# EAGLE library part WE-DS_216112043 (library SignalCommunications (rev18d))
WE-DS D-SUB-Filter Connectors Bent 90° Characteristics Standard type filtered with 1000 pF High attenuation of more than 40 dB @ 180 MHz Choice of earthing metal sheet or high speed earthing clip Rated voltage: 100 VDC Rated current @ 20 ºC: 5 A Withstand voltage: 250 VRMS Insulation resistance: min. 1000 MΩ Operating temperature: –55 ºC to +125 ºC Applications Filtering of interfaces External connection to -printer -sensor -display Details see: http://katalog.we-online.de/en/pbs/Filter_abgewinkelt Created on 2015-05-04 2015 (C) Wurth Elektronik
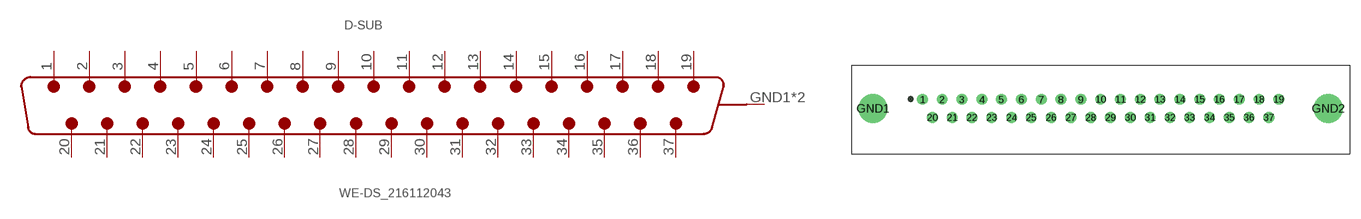
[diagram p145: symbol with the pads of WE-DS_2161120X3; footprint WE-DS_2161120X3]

Designator prefix D-SUB

## WE-DS_216112043 (WE-NUMBER: 216112043/37Pins_male)  [WE-DS_2161120X3]
1  1  pas
2  2  pas
3  3  pas
4  4  pas
5  5  pas
6  6  pas
7  7  pas
8  8  pas
9  9  pas
10  10  pas
11  11  pas
12  12  pas
13  13  pas
14  14  pas
15  15  pas
16  16  pas
17  17  pas
18  18  pas
19  19  pas
20  20  pas
21  21  pas
22  22  pas
23  23  pas
24  24  pas
25  25  pas
26  26  pas
27  27  pas
28  28  pas
29  29  pas
30  30  pas
31  31  pas
32  32  pas
33  33  pas
34  34  pas
35  35  pas
36  36  pas
37  37  pas
GND1  GND  pwr
GND2  GND  pwr

## Footprint WE-DS_2161120X3 (pad centres in mm)
drill 1: 1 -24.84,1.27; 2 -22.1,1.27; 3 -19.33,1.27; 4 -16.56,1.27; 5 -13.82,1.27; 6 -11.05,1.27; 7 -8.28,1.27; 8 -5.54,1.27; 9 -2.77,1.27; 10 0,1.27; 11 2.77,1.27; 12 5.54,1.27; 13 8.28,1.27; 14 11.05,1.27; 15 13.82,1.27; 16 16.56,1.27; 17 19.33,1.27; 18 22.1,1.27; 19 24.84,1.27; 20 -23.47,-1.27; 21 -20.7,-1.27; 22 -17.96,-1.27; 23 -15.19,-1.27; 24 -12.42,-1.27; 25 -9.68,-1.27; 26 -6.91,-1.27; 27 -4.14,-1.27; 28 -1.38,-1.27; 29 1.38,-1.27; 30 4.14,-1.27; 31 6.91,-1.27; 32 9.68,-1.27; 33 12.42,-1.27; 34 15.19,-1.27; 35 17.96,-1.27; 36 20.7,-1.27; 37 23.47,-1.27
drill 3: GND1 -31.75,0; GND2 31.75,0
